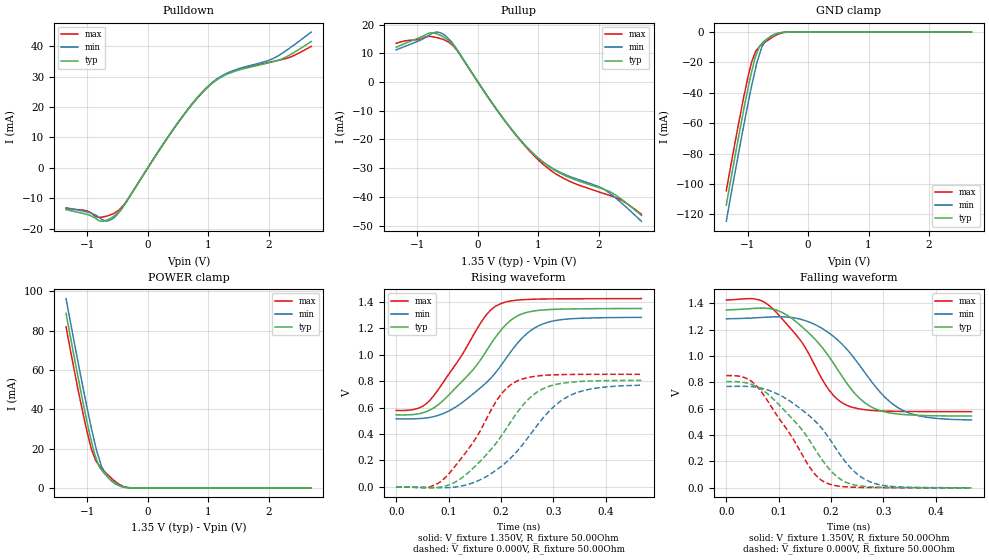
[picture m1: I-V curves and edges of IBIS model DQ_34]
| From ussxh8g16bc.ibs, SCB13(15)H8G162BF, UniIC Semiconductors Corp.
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| MODEL DQ_34 (34 Ohm Data I/O with no ODT, 800-2133Mbps)
[Model]   DQ_34
Model_type   I/O
Vinl = 545.000mV
Vinh = 805.000mV
Vmeas = 675.000mV
Vref = 675.000mV
Cref = 0.0pF
Rref = 25.000Ohm
|   typ   min   max
|C_comp   0.950pF   0.900pF   1.000pF
C_comp_pullup   0.4750pF   0.4500pF   0.5000pF
C_comp_pulldown   0.4750pF   0.4500pF   0.5000pF
[Model Spec]
| Input threshold voltage corners
Vinl   0.5450V   0.5115V   0.5825V
Vinh   0.8050V   0.7715V   0.8425V
| Measurement voltage corners
Vmeas   0.6750V   0.6415V   0.7125V
| Timing spec test load voltage corners
Vref   0.6750V   0.6415V   0.7125V
| Dynamic Overshoot Parameters from DDR3L Specification
|D_overshoot_ampl_h   0.40   NA   NA
|D_overshoot_ampl_l   0.40   NA   NA
|D_overshoot_area_h   0.11n   NA   NA
|D_overshoot_area_l   0.11n   NA   NA
[Receiver Thresholds]
Vth   =  0.675V
Vth_min  =  0.6615V
Vth_max  =  0.6885V
Vinh_ac  =  0.130V
Vinh_dc  =  0.090V
Vinl_ac  = -0.130V
Vinl_dc  = -0.090V
Tslew_ac =  5.000ns |Not specified, so set to high value
Threshold_sensitivity = 0.50
Reference_supply Pullup_ref
[Voltage Range]   1.3500V   1.2830V   1.4250V
[Pullup Reference]   1.3500V   1.2830V   1.4250V
| Junction Temperature (Ambient temp is 40C typ, 85C min, 0C max)
[Temperature Range]   45.0   90.0   0.0
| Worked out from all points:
|   slope of the pulldown table from 0 to 0.203 V, typ, clamps not added: 32.4 ohm
|   slope of the pullup table from 0 to 0.203 V, typ, clamps not added: 32.1 ohm
|   GND clamp passes 1 mA (typ) near -0.50 V on its own axis
|   POWER clamp passes 1 mA (typ) near -0.45 V on its own axis
|   falling waveform, V_fixture 1.350V, R_fixture 50.00Ohm: 20-80 % time 94.1ps typ, 97.5ps min, 82.7ps max; typ from 1.35 V to 0.545 V
|   rising waveform, V_fixture 1.350V, R_fixture 50.00Ohm: 20-80 % time 97.7ps typ, 105ps min, 81.4ps max; typ from 0.545 V to 1.35 V
|   rising waveform, V_fixture 0.000V, R_fixture 50.00Ohm: 20-80 % time 95.5ps typ, 103ps min, 81.4ps max; typ from 0 V to 0.806 V
|   falling waveform, V_fixture 0.000V, R_fixture 50.00Ohm: 20-80 % time 95.4ps typ, 100ps min, 81.6ps max; typ from 0.806 V to 0 V
[Pulldown]
|   Voltage   I(typ)   I(min)   I(max)
-1.35V    -13.75mA   -13.12mA   -13.4mA
-1V       -15.34mA   -14.53mA   -14.16mA
-800mV    -17.5mA    -16.38mA   -16.3mA
-690mV    -17.29mA   -17.5mA    -15.92mA
-565mV    -15.95mA   -16.5mA    -15.03mA
-395mV    -12.31mA   -12.44mA   -12.15mA
560mV     16.52mA    16.6mA     16.45mA
1.055V    27.67mA    27.92mA    27.71mA
1.465V    31.94mA    32.36mA    32.16mA
2.105V    35.05mA    36.27mA    35.14mA
2.34V     37.07mA    39.31mA    36.32mA
2.7V      41.52mA    44.64mA    39.91mA
[GND Clamp]
|   Voltage   I(typ)   I(min)   I(max)
-1.35V    -113.9mA   -124.6mA   -104.5mA
-1.205V   -81.48mA   -92.16mA   -72.46mA
-1.07V    -52.65mA   -63.14mA   -44.3mA
-1V       -38.7mA    -48.81mA   -30.85mA
-930mV    -25.95mA   -35.02mA   -19.4mA
-875mV    -16.88mA   -25.36mA   -13.69mA
-800mV    -9.222mA   -14.41mA   -9.487mA
-765mV    -7.604mA   -9.974mA   -8.359mA
-650mV    -3.918mA   -3.687mA   -5.017mA
-520mV    -1.303mA   -937.1uA   -1.955mA
-315mV    -19.67uA   -18.79uA   -28.64uA
2.7V      0A         0A         0A
[Pullup]
|   Voltage   I(typ)   I(min)   I(max)
-1.35V    12.15mA    11.27mA    13.53mA
-800mV    17.18mA    16.42mA    15.95mA
-690mV    16.9mA     17.47mA    15.58mA
-565mV    15.71mA    16.61mA    14.82mA
-320mV    10.4mA     10.58mA    10.31mA
470mV     -14.09mA   -14.2mA    -14.2mA
775mV     -21.88mA   -21.96mA   -22.19mA
1.055V    -27.57mA   -27.49mA   -28.24mA
1.465V    -32.85mA   -32.46mA   -34.09mA
2.105V    -37.57mA   -37.65mA   -39.03mA
2.34V     -40.35mA   -41.55mA   -40.81mA
2.7V      -46.46mA   -48.53mA   -46.05mA
[POWER Clamp]
|   Voltage   I(typ)   I(min)   I(max)
-1.35V    88.89mA    96.37mA    82.02mA
-1.205V   64.87mA    72.5mA     58.31mA
-1.07V    43.46mA    51mA       37.77mA
-930mV    23.58mA    30.09mA    19.57mA
-875mV    16.77mA    22.82mA    15.04mA
-800mV    10.68mA    14.43mA    11.22mA
-765mV    9.147mA    10.97mA    10.01mA
-690mV    6.433mA    6.617mA    7.571mA
-565mV    3.162mA    2.653mA    3.926mA
-395mV    485.8uA    358.5uA    537uA
-310mV    60.31uA    60.42uA    66.72uA
2.7V      0A         0A         0A
[Ramp]
R_load = 50.00Ohm
|   typ   min   max
dV/dt_r   483.363mV/95.498ps  461.741mV/103.129ps 511.044mV/81.416ps
dV/dt_f   483.183mV/94.118ps  460.840mV/97.492ps  508.075mV/82.746ps
[Falling Waveform]
V_fixture = 1.350V
V_fixture_min = 1.283V
V_fixture_max = 1.425V
R_fixture = 50.00Ohm
|   Time   V(typ)   V(min)   V(max)
0s        1.35V      1.283V     1.425V
54ps      1.362V     1.29V      1.434V
84ps      1.359V     1.296V     1.375V
162ps     1.157V     1.252V     983.3mV
198ps     984.4mV    1.169V     731.9mV
230ps     793.7mV    1.052V     626.7mV
274ps     620mV      823mV      588.6mV
328ps     560.3mV    607.7mV    580.3mV
382ps     548.1mV    535.9mV    578.6mV
468ps     544.7mV    514.9mV    578.2mV
[Rising Waveform]
V_fixture = 1.350V
V_fixture_min = 1.283V
V_fixture_max = 1.425V
R_fixture = 50.00Ohm
|   Time   V(typ)   V(min)   V(max)
0s        544.7mV    514.9mV    578.2mV
38ps      549.8mV    515.5mV    589.7mV
64ps      581mV      525.1mV    654.1mV
122ps     783.2mV    626.6mV    976.2mV
168ps     1.004V     774.3mV    1.281V
198ps     1.176V     907.7mV    1.384V
232ps     1.295V     1.089V     1.414V
280ps     1.339V     1.233V     1.422V
336ps     1.347V     1.273V     1.424V
468ps     1.35V      1.283V     1.425V
[Rising Waveform]
V_fixture = 0.000V
V_fixture_min = 0.000V
V_fixture_max = 0.000V
R_fixture = 50.00Ohm
|   Time   V(typ)   V(min)   V(max)
0s        -7.022uV   -2.894uV   8.479uV
58ps      -6.88mV    -4.479mV   -4.015mV
90ps      2.398mV    -6.977mV   56.33mV
158ps     184.2mV    49.04mV    407.1mV
198ps     369.9mV    147.2mV    688.6mV
230ps     558mV      266mV      799.2mV
274ps     729.5mV    490.1mV    841.1mV
328ps     789.7mV    683.7mV    850.4mV
382ps     802.6mV    747.6mV    851.9mV
468ps     805.6mV    769.6mV    851.7mV
[Falling Waveform]
V_fixture = 0.000V
V_fixture_min = 0.000V
V_fixture_max = 0.000V
R_fixture = 50.00Ohm
|   Time   V(typ)   V(min)   V(max)
0s        805.6mV    769.6mV    851.7mV
44ps      790.3mV    769.1mV    818.7mV
80ps      709.5mV    741mV      652.6mV
136ps     480.7mV    616.9mV    313.1mV
162ps     340mV      534.4mV    139.5mV
190ps     174.4mV    411.4mV    38.77mV
224ps     50.86mV    214.1mV    8.638mV
274ps     7.338mV    46.17mV    2.195mV
328ps     1.954mV    7.099mV    1.08mV
468ps     -7.022uV   -2.894uV   8.479uV
